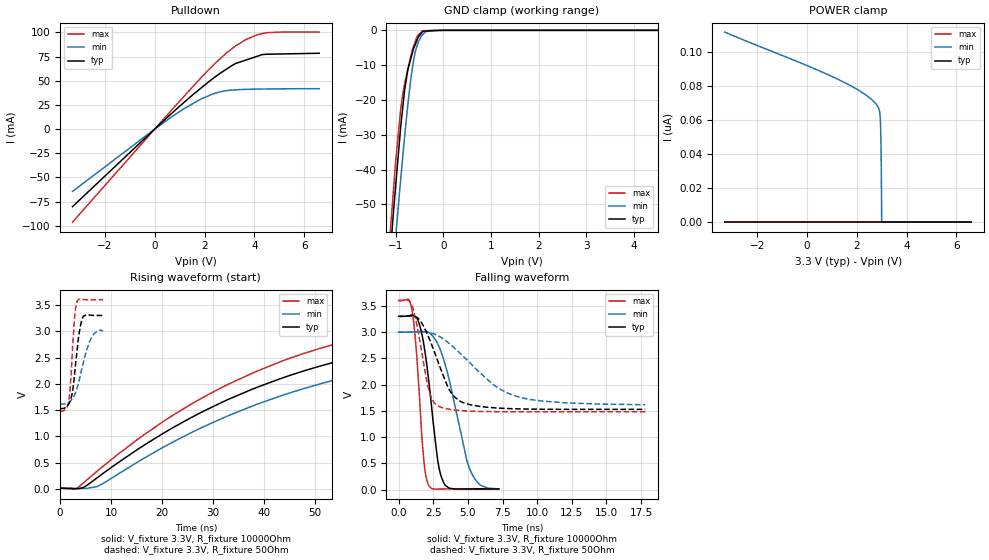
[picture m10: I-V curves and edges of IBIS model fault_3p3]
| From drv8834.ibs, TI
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|   fault_3p3 Model
[Model]   fault_3p3
Model_type   Open_drain
Polarity   Inverting
Vmeas = 1.65
Vref = 3.3
Cref = 2pF
Rref = 10000
|   typ   min   max
|   (nom PVT)   (fast PVT)   (slow PVT)
|C_comp from frequency sweep method (F=125KHz)
|C_comp   9.084e-12   3.182e-13   1.609e-11
|ON state : BUFFER OUTPUT TURNED LOW
|C_comp   9.084e-12   3.182e-13   1.609e-11
|OFF state: BUFFER IN HIGH IMPEDANCE
|C_comp   3.668e-12   3.444e-12   3.902e-12
|C_comp from LC tank measurement(L=1nH)
|Resonant Frequency(Hz)   3.910e+09   3.950e+09   3.720e+09
 C_comp   1.659e-12   1.625e-12   1.832e-12
|ON state : BUFFER OUTPUT TURNED LOW
|Resonant Frequency(Hz)   3.910e+09   3.950e+09   3.720e+09
|C_comp   1.659e-12   1.625e-12   1.832e-12
|OFF state: BUFFER IN HIGH IMPEDANCE
|Resonant Frequency(Hz)   3.270e+09   3.320e+09   3.190e+09
|C_comp   2.371e-12   2.300e-12   2.492e-12
| Where nom  PVT is Nominal Process, 3.3V, 27C
|   Fast PVT is Strong Process,  3.6V, -40C
|   Slow PVT is Weak Process,   3V, 125C
[Voltage Range]   3.3   3   3.6
|Ambient Temperature   25   150   -40
|Junction Temperature
[Temperature Range]   27   125   -40
[Pullup Reference]   3.3   3   3.6
[Pulldown Reference]   0   0   0
[Power Clamp Reference]   3.3   3   3.6
[GND Clamp Reference]   0   0   0
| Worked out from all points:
|   slope of the pulldown table from 0 to 0.495 V, typ, clamps not added: 41.8 ohm
|   GND clamp passes 1 mA (typ) near -0.47 V on its own axis
|   falling waveform, V_fixture 3.3V, R_fixture 10000Ohm: 20-80 % time 874ps typ, 1.54ns min, 559ps max; typ from 3.3 V to 0.015 V
|   rising waveform, V_fixture 3.3V, R_fixture 10000Ohm: 20-80 % time 49.7ns typ, 52.5ns min, 46.4ns max; typ from 0.014 V to 3.3 V
|   falling waveform, V_fixture 3.3V, R_fixture 50Ohm: 20-80 % time 1.6ns typ, 3.55ns min, 884ps max; typ from 3.3 V to 1.53 V
|   rising waveform, V_fixture 3.3V, R_fixture 50Ohm: 20-80 % time 1.23ns typ, 2.28ns min, 813ps max; typ from 1.53 V to 3.3 V
[Pulldown]
|   Voltage   I(typ)   I(min)   I(max)
-3.3V     -80.18mA   -64.45mA   -96.25mA
18mV      435.3uA    350.4uA    525uA
1.143V    26.89mA    20.57mA    32.98mA
1.764V    40.47mA    29.81mA    50.49mA
2.301V    51.58mA    36.01mA    64.84mA
2.658V    58.25mA    38.76mA    73.54mA
3.089V    65.52mA    40.36mA    82.96mA
3.241V    67.79mA    40.6mA     85.83mA
3.661V    71.41mA    41.1mA     92.57mA
4.316V    77.05mA    41.45mA    98.84mA
5.058V    77.69mA    41.63mA    100.3mA
6.6V      78.43mA    41.85mA    100.3mA
[GND Clamp]
|   Voltage   I(typ)   I(min)   I(max)
-3.3V     -509.7mA   -494.9mA   -536mA
-1.134V   -67.38mA   -80.8mA    -60.88mA
-1.077V   -57.22mA   -71.32mA   -50.79mA
-1.001V   -44.33mA   -59.19mA   -37.31mA
-896.4mV  -27.62mA   -42.57mA   -22.5mA
-818.4mV  -17.5mA    -31.08mA   -15.66mA
-745.8mV  -11.18mA   -21.2mA    -11.11mA
-684mV    -8.091mA   -13.91mA   -7.337mA
-591mV    -4.04mA    -6.22mA    -3.227mA
-442.8mV  -484.8uA   -1.345mA   -159.5uA
-153mV    -79.11uA   -3.863uA   -9.382uA
6.6V      0A         0A         0A
[POWER Clamp]
|   Voltage   I(typ)   I(min)   I(max)
-3.3V     0A         111.8nA    0A
1.167V    0A         84.58nA    0A
2.32V     0A         75.26nA    0A
2.772V    0A         69.5nA     0A
2.907V    0A         65.57nA    0A
2.946V    0A         59.82nA    0A
2.961V    0A         52.86nA    0A
2.976V    0A         39.55nA    0A
2.985V    0A         27.57nA    0A
2.994V    0A         12.21nA    0A
2.997V    0A         0A         0A
6.6V      0A         0A         0A
[Ramp]
R_load = 10000
|   typ   min   max
dV/dt_r   1.97187/4.98681e-08   1.79025/5.2736e-08   2.15262/4.64947e-08
dV/dt_f   1.97187/8.74014e-10   1.79025/1.54127e-09   2.15262/5.58491e-10
[Falling Waveform]
V_fixture = 3.3V
V_fixture_min = 3V
V_fixture_max = 3.6V
R_fixture = 10000Ohm
C_fixture = 0F
|   Time   V(typ)   V(min)   V(max)
0s        3.3V       2.999V     3.6V
700ps     3.311V     2.999V     3.629V
975ps     3.324V     3.003V     3.409V
1.275ns   3.278V     3.009V     2.658V
1.825ns   2.755V     3.012V     548.3mV
2.175ns   2.072V     2.994V     77.73mV
2.8ns     598.3mV    2.791V     12.32mV
3.325ns   100.4mV    2.413V     15.44mV
5.2ns     16.3mV     352.5mV    13.46mV
7.225ns   15.36mV    15.96mV    12.34mV
[Rising Waveform]
V_fixture = 3.3V
V_fixture_min = 3V
V_fixture_max = 3.6V
R_fixture = 10000Ohm
C_fixture = 0F
|   Time   V(typ)   V(min)   V(max)
0s        13.53mV    15.33mV    12.3mV
3.3ns     3.355mV    8.664mV    11.1mV
7.225ns   207.4mV    43.46mV    334mV
22.03ns   1.16V      886.4mV    1.396V
37.55ns   1.892V     1.571V     2.195V
55.1ns    2.446V     2.105V     2.789V
72.4ns    2.793V     2.445V     3.144V
96.5ns    3.064V     2.72V      3.404V
124.9ns   3.198V     2.872V     3.521V
225.4ns   3.297V     2.993V     3.598V
[Falling Waveform]
V_fixture = 3.3V
V_fixture_min = 3V
V_fixture_max = 3.6V
R_fixture = 50Ohm
C_fixture = 0F
|   Time   V(typ)   V(min)   V(max)
0s        3.3V       3V         3.6V
950ps     3.308V     3.001V     3.516V
1.55ns    3.219V     3.003V     2.805V
2.2ns     2.884V     2.994V     1.878V
2.95ns    2.358V     2.917V     1.581V
3.625ns   1.917V     2.79V      1.534V
4.45ns    1.684V     2.595V     1.507V
6.9ns     1.559V     1.989V     1.486V
8.15ns    1.543V     1.81V      1.485V
17.8ns    1.53V      1.618V     1.484V
[Rising Waveform]
V_fixture = 3.3V
V_fixture_min = 3V
V_fixture_max = 3.6V
R_fixture = 50Ohm
C_fixture = 0F
|   Time   V(typ)   V(min)   V(max)
0s        1.527V     1.613V     1.477V
1ns       1.544V     1.619V     1.511V
1.675ns   1.614V     1.646V     1.657V
2.075ns   1.698V     1.678V     2.074V
2.8ns     2.148V     1.78V      3.233V
3.325ns   2.639V     1.92V      3.569V
3.85ns    3.033V     2.114V     3.612V
4.5ns     3.274V     2.38V      3.604V
6.225ns   3.303V     2.893V     3.6V
8.4ns     3.3V       3.008V     3.6V
